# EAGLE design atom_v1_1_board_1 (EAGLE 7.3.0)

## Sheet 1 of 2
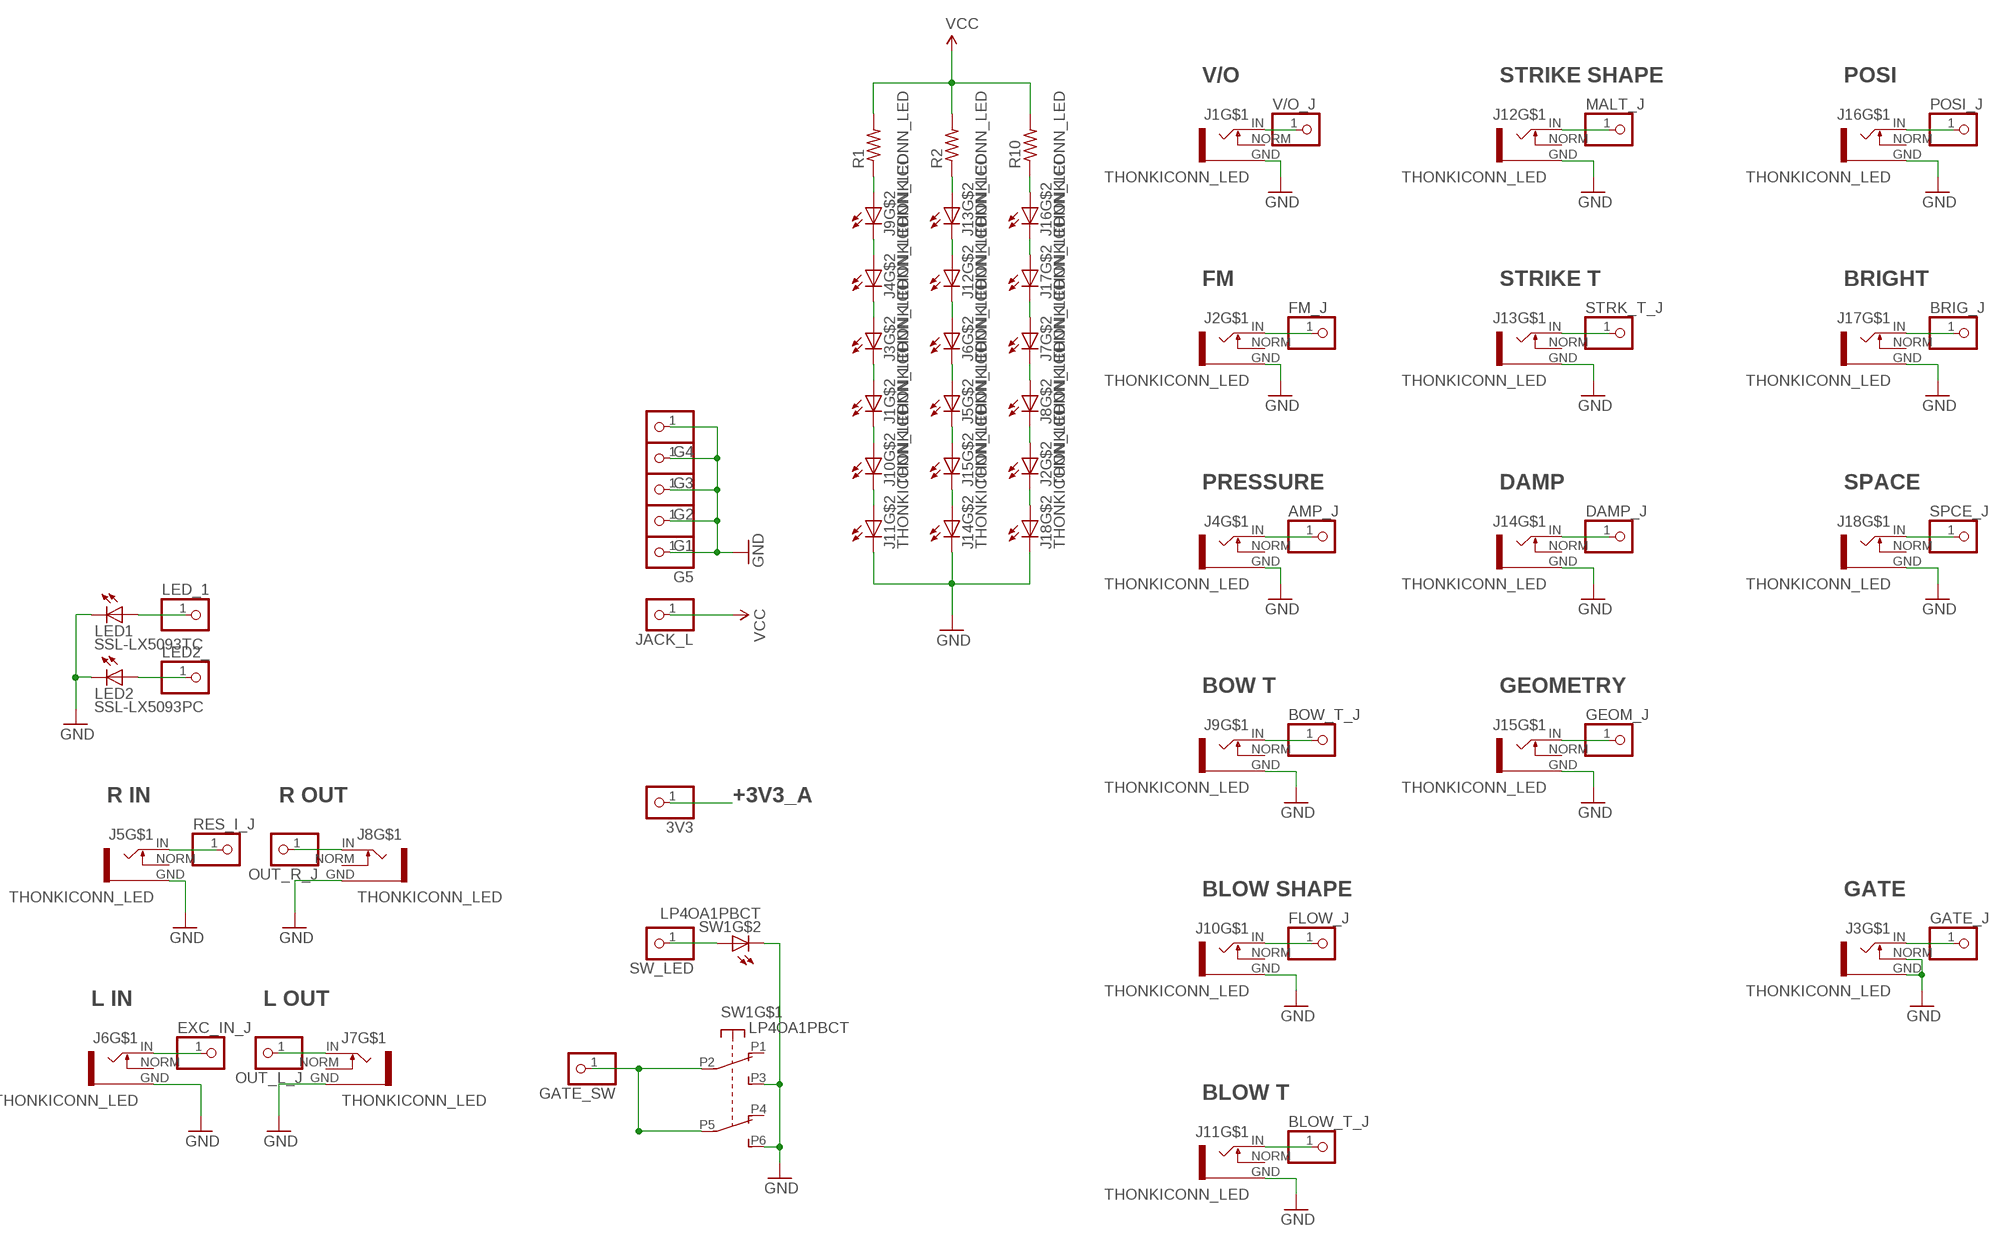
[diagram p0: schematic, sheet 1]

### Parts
3V3  PINHD-1X1  [1X01]
AMP_J  PINHD-1X1  [1X01]
BLOW_T_J  PINHD-1X1  [1X01]
BOW_T_J  PINHD-1X1  [1X01]
BRIG_J  PINHD-1X1  [1X01]
DAMP_J  PINHD-1X1  [1X01]
EXC_IN_J  PINHD-1X1  [1X01]
FLOW_J  PINHD-1X1  [1X01]
FM_J  PINHD-1X1  [1X01]
G1  PINHD-1X1  [1X01]
G2  PINHD-1X1  [1X01]
G3  PINHD-1X1  [1X01]
G4  PINHD-1X1  [1X01]
G5  PINHD-1X1  [1X01]
GATE_J  PINHD-1X1  [1X01]
GATE_SW  PINHD-1X1  [1X01]
GEOM_J  PINHD-1X1  [1X01]
J1  THONKICONN_LED  [LED_JACK]
J2  THONKICONN_LED  [LED_JACK]
J3  THONKICONN_LED  [LED_JACK]
J4  THONKICONN_LED  [LED_JACK]
J5  THONKICONN_LED  [LED_JACK]
J6  THONKICONN_LED  [LED_JACK]
J7  THONKICONN_LED  [LED_JACK]
J8  THONKICONN_LED  [LED_JACK]
J9  THONKICONN_LED  [LED_JACK]
J10  THONKICONN_LED  [LED_JACK]
J11  THONKICONN_LED  [LED_JACK]
J12  THONKICONN_LED  [LED_JACK]
J13  THONKICONN_LED  [LED_JACK]
J14  THONKICONN_LED  [LED_JACK]
J15  THONKICONN_LED  [LED_JACK]
J16  THONKICONN_LED  [LED_JACK]
J17  THONKICONN_LED  [LED_JACK]
J18  THONKICONN_LED  [LED_JACK]
JACK_L  PINHD-1X1  [1X01]
LED1  SSL-LX5093TC  LED5MM  [LED_5MM]
LED2  SSL-LX5093PC  LED5MM  [LED_5MM]
LED2_  PINHD-1X1  [1X01]
LED_1  PINHD-1X1  [1X01]
MALT_J  PINHD-1X1  [1X01]
OUT_L_J  PINHD-1X1  [1X01]
OUT_R_J  PINHD-1X1  [1X01]
POSI_J  PINHD-1X1  [1X01]
R1  RESISTOR  [RESISTOR_0603]
R2  RESISTOR  [RESISTOR_0603]
R10  RESISTOR  [RESISTOR_0603]
RES_I_J  PINHD-1X1  [1X01]
SPCE_J  PINHD-1X1  [1X01]
STRK_T_J  PINHD-1X1  [1X01]
SW1  LP4OA1PBCT  [LP4OA1PBCT]
SW_LED  PINHD-1X1  [1X01]
V/O_J  PINHD-1X1  [1X01]

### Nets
+3V3_A: 3V3.1 ; also sheet 2
GND: G1.1 G2.1 G3.1 G4.1 G5.1 J1.GND J2.GND J3.GND J3.NORM J4.GND J5.GND J6.GND J7.GND J8.GND J9.GND J10.GND J11.C J11.GND J12.GND J13.GND J14.C J14.GND J15.GND J16.GND J17.GND J18.C J18.GND LED1.K(C) LED2.K(C) SW1.L2 SW1.P3(A3) SW1.P6(B3) ; also sheet 2
N$1: J1.IN V/O_J.1
N$3: J12.IN MALT_J.1
N$4 [wide]: J9.A R1.1
N$5 [wide]: J4.A J9.C
N$6: FM_J.1 J2.IN
N$7 [wide]: J3.A J4.C
N$8 [wide]: J1.A J3.C
N$9 [wide]: J1.C J10.A
N$10 [wide]: J10.C J11.A
N$12: J13.IN STRK_T_J.1
N$13 [wide]: J2.C J18.A
N$14 [wide]: J2.A J8.C
N$15 [wide]: J7.C J8.A
N$16: DAMP_J.1 J14.IN
N$17 [wide]: J7.A J17.C
N$18 [wide]: J16.C J17.A
N$19 [wide]: J16.A R10.1
N$20: J5.IN RES_I_J.1
N$21: EXC_IN_J.1 J6.IN
N$22 [wide]: J13.A R2.1
N$23 [wide]: J12.A J13.C
N$24 [wide]: J6.A J12.C
N$25 [wide]: J5.A J6.C
N$26: AMP_J.1 J4.IN
N$27 [wide]: J5.C J15.A
N$28 [wide]: J14.A J15.C
N$29: J16.IN POSI_J.1
N$34: BRIG_J.1 J17.IN
N$36: GEOM_J.1 J15.IN
N$39: J18.IN SPCE_J.1
N$43: GATE_J.1 J3.IN
N$59: LED1.A LED_1.1
N$60: LED2.A LED2_.1
N$83: J8.IN OUT_R_J.1
N$85: J7.IN OUT_L_J.1
N$90: BOW_T_J.1 J9.IN
N$91: FLOW_J.1 J10.IN
N$92: BLOW_T_J.1 J11.IN
N$128: SW1.L1 SW_LED.1
SW_GATE: GATE_SW.1 SW1.P2(A2) SW1.P5(B2)
VCC [wide]: JACK_L.1 R1.2 R2.2 R10.2
Unconnected: J1.NORM J2.NORM J4.NORM J5.NORM J6.NORM J7.NORM J8.NORM J9.NORM J10.NORM J11.NORM J12.NORM J13.NORM J14.NORM J15.NORM J16.NORM J17.NORM J18.NORM SW1.P1(A1) SW1.P4(B1)

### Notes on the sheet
- V/O | STRIKE SHAPE | POSI
- FM | STRIKE T | BRIGHT
- PRESSURE | DAMP | SPACE
- BOW T | GEOMETRY
- R IN | R OUT
- BLOW SHAPE | GATE
- L IN | L OUT
- BLOW T

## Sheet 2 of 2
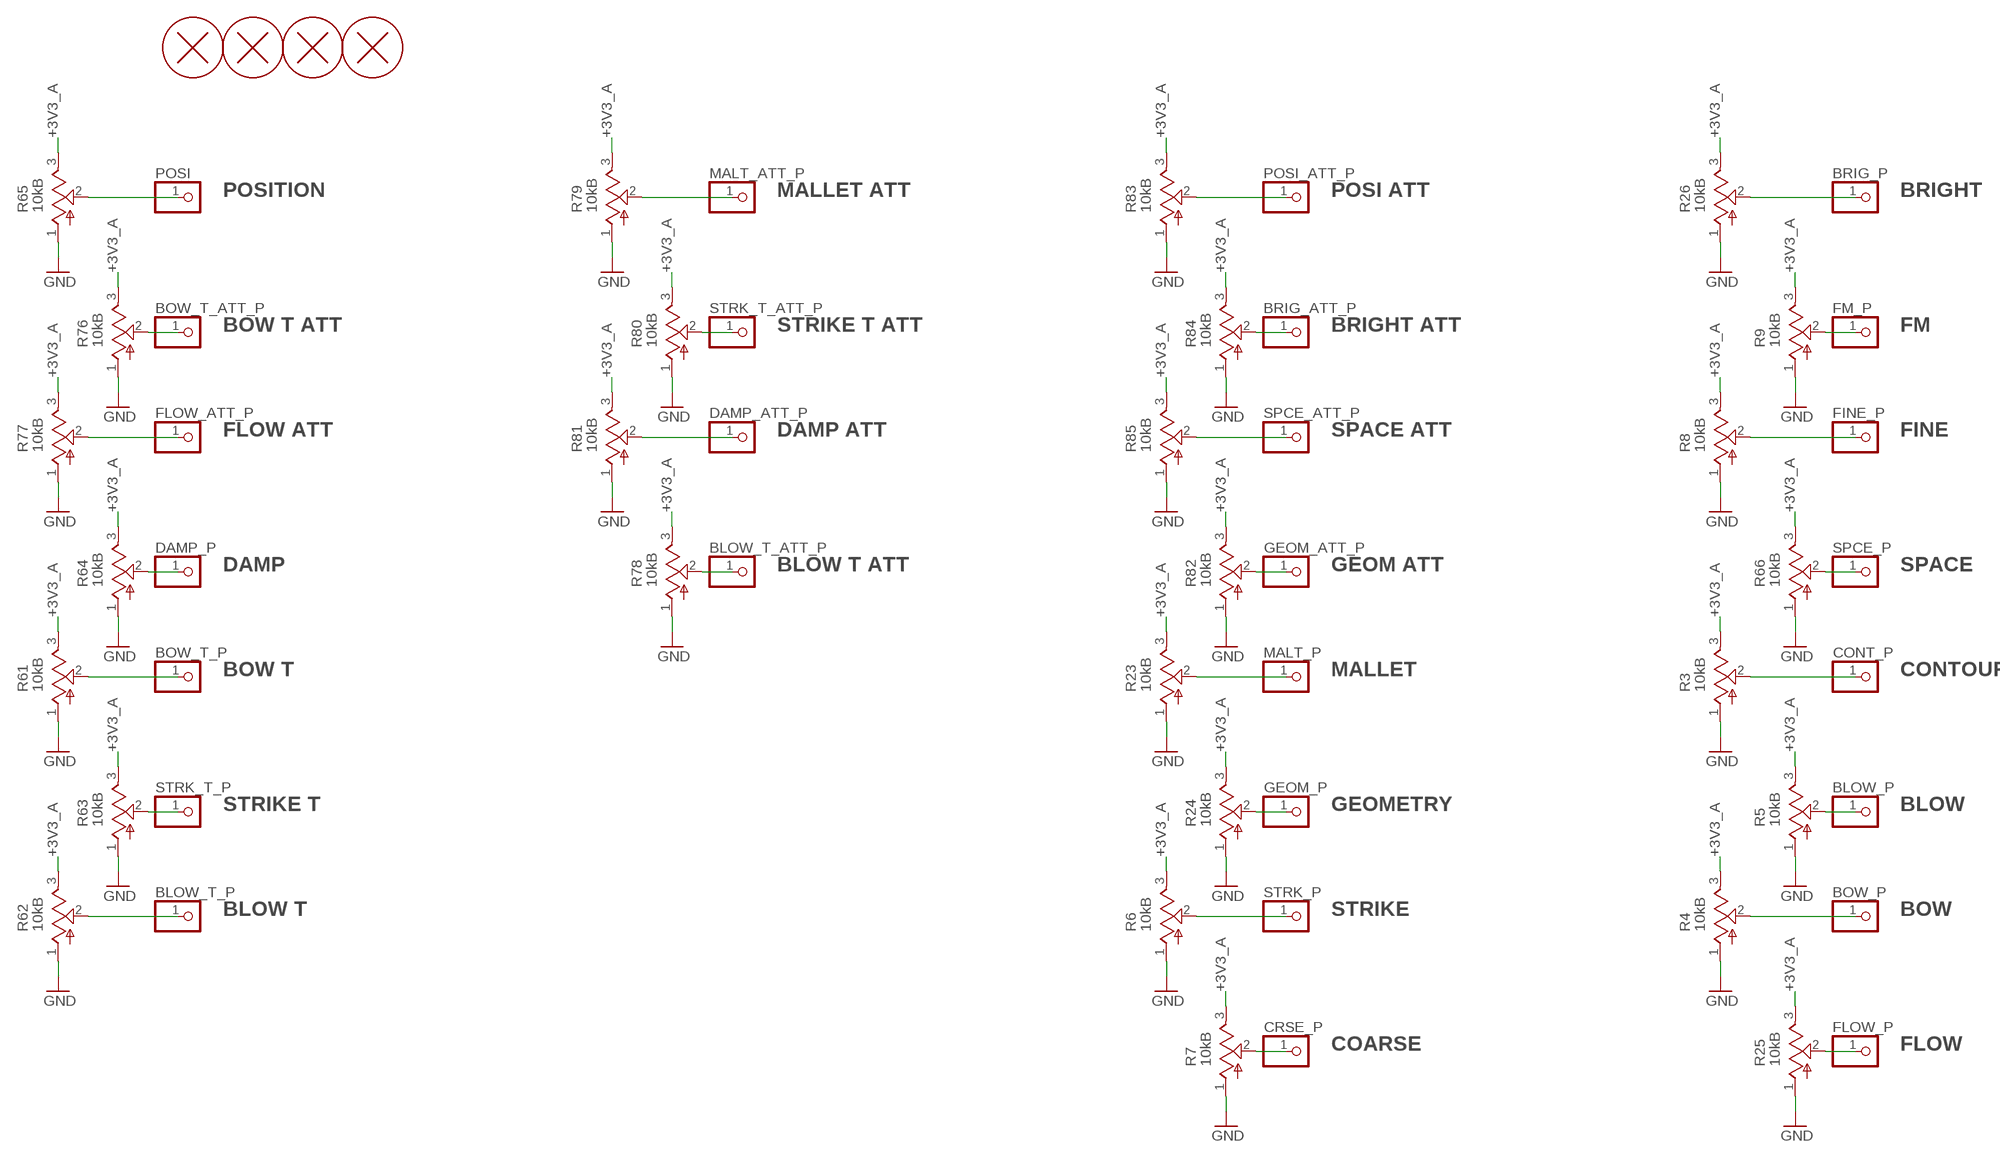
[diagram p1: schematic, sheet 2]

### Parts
BLOW_P  PINHD-1X1  [1X01]
BLOW_T_ATT_P  PINHD-1X1  [1X01]
BLOW_T_P  PINHD-1X1  [1X01]
BOW_P  PINHD-1X1  [1X01]
BOW_T_ATT_P  PINHD-1X1  [1X01]
BOW_T_P  PINHD-1X1  [1X01]
BRIG_ATT_P  PINHD-1X1  [1X01]
BRIG_P  PINHD-1X1  [1X01]
CONT_P  PINHD-1X1  [1X01]
CRSE_P  PINHD-1X1  [1X01]
DAMP_ATT_P  PINHD-1X1  [1X01]
DAMP_P  PINHD-1X1  [1X01]
FINE_P  PINHD-1X1  [1X01]
FLOW_ATT_P  PINHD-1X1  [1X01]
FLOW_P  PINHD-1X1  [1X01]
FM_P  PINHD-1X1  [1X01]
GEOM_ATT_P  PINHD-1X1  [1X01]
GEOM_P  PINHD-1X1  [1X01]
H1  PCB_SCREW  [PCB_SCREW]
H2  PCB_SCREW  [PCB_SCREW]
H3  PCB_SCREW  [PCB_SCREW]
H4  PCB_SCREW  [PCB_SCREW]
MALT_ATT_P  PINHD-1X1  [1X01]
MALT_P  PINHD-1X1  [1X01]
POSI  PINHD-1X1  [1X01]
POSI_ATT_P  PINHD-1X1  [1X01]
R3  10kB  POT_VERTICAL  [ALPS_POT_VERTICAL]
R4  10kB  POT_VERTICAL  [ALPS_POT_VERTICAL]
R5  10kB  POT_VERTICAL  [ALPS_POT_VERTICAL]
R6  10kB  POT_VERTICAL  [ALPS_POT_VERTICAL]
R7  10kB  POT_VERTICAL  [ALPS_POT_VERTICAL]
R8  10kB  POT_VERTICAL  [ALPS_POT_VERTICAL]
R9  10kB  POT_VERTICAL  [ALPS_POT_VERTICAL]
R23  10kB  POT_VERTICAL  [ALPS_POT_VERTICAL]
R24  10kB  POT_VERTICAL  [ALPS_POT_VERTICAL]
R25  10kB  POT_VERTICAL  [ALPS_POT_VERTICAL]
R26  10kB  POT_VERTICAL  [ALPS_POT_VERTICAL]
R61  10kB  POT_VERTICAL  [ALPS_POT_VERTICAL]
R62  10kB  POT_VERTICAL  [ALPS_POT_VERTICAL]
R63  10kB  POT_VERTICAL  [ALPS_POT_VERTICAL]
R64  10kB  POT_VERTICAL  [ALPS_POT_VERTICAL]
R65  10kB  POT_VERTICAL  [ALPS_POT_VERTICAL]
R66  10kB  POT_VERTICAL  [ALPS_POT_VERTICAL]
R76  10kB  POT_VERTICAL  [ALPS_POT_VERTICAL]
R77  10kB  POT_VERTICAL  [ALPS_POT_VERTICAL]
R78  10kB  POT_VERTICAL  [ALPS_POT_VERTICAL]
R79  10kB  POT_VERTICAL  [ALPS_POT_VERTICAL]
R80  10kB  POT_VERTICAL  [ALPS_POT_VERTICAL]
R81  10kB  POT_VERTICAL  [ALPS_POT_VERTICAL]
R82  10kB  POT_VERTICAL  [ALPS_POT_VERTICAL]
R83  10kB  POT_VERTICAL  [ALPS_POT_VERTICAL]
R84  10kB  POT_VERTICAL  [ALPS_POT_VERTICAL]
R85  10kB  POT_VERTICAL  [ALPS_POT_VERTICAL]
SPCE_ATT_P  PINHD-1X1  [1X01]
SPCE_P  PINHD-1X1  [1X01]
STRK_P  PINHD-1X1  [1X01]
STRK_T_ATT_P  PINHD-1X1  [1X01]
STRK_T_P  PINHD-1X1  [1X01]

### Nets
+3V3_A: R3.3(B) R4.3(B) R5.3(B) R6.3(B) R7.3(B) R8.3(B) R9.3(B) R23.3(B) R24.3(B) R25.3(B) R26.3(B) R61.3(B) R62.3(B) R63.3(B) R64.3(B) R65.3(B) R66.3(B) R76.3(B) R77.3(B) R78.3(B) R79.3(B) R80.3(B) R81.3(B) R82.3(B) R83.3(B) R84.3(B) R85.3(B) ; also sheet 1
GND: R3.1(A) R4.1(A) R5.1(A) R6.1(A) R7.1(A) R8.1(A) R9.1(A) R23.1(A) R24.1(A) R25.1(A) R26.1(A) R61.1(A) R62.1(A) R63.1(A) R64.1(A) R65.1(A) R66.1(A) R76.1(A) R77.1(A) R78.1(A) R79.1(A) R80.1(A) R81.1(A) R82.1(A) R83.1(A) R84.1(A) R85.1(A) ; also sheet 1
N$45: BOW_T_ATT_P.1 R76.2(W)
N$46: POSI.1 R65.2(W)
N$47: MALT_ATT_P.1 R79.2(W)
N$48: DAMP_P.1 R64.2(W)
N$49: BOW_T_P.1 R61.2(W)
N$50: R80.2(W) STRK_T_ATT_P.1
N$51: BLOW_T_ATT_P.1 R78.2(W)
N$52: R63.2(W) STRK_T_P.1
N$53: BLOW_T_P.1 R62.2(W)
N$55: FLOW_ATT_P.1 R77.2(W)
N$57: DAMP_ATT_P.1 R81.2(W)
N$58: R85.2(W) SPCE_ATT_P.1
N$62: BRIG_P.1 R26.2(W)
N$63: FINE_P.1 R8.2(W)
N$65: GEOM_ATT_P.1 R82.2(W)
N$67: CRSE_P.1 R7.2(W)
N$68: FM_P.1 R9.2(W)
N$69: R6.2(W) STRK_P.1
N$70: GEOM_P.1 R24.2(W)
N$71: MALT_P.1 R23.2(W)
N$72: FLOW_P.1 R25.2(W)
N$73: BOW_P.1 R4.2(W)
N$74: CONT_P.1 R3.2(W)
N$75: BLOW_P.1 R5.2(W)
N$76: POSI_ATT_P.1 R83.2(W)
N$77: BRIG_ATT_P.1 R84.2(W)
N$78: R66.2(W) SPCE_P.1

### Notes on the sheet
- POSITION | MALLET ATT | POSI ATT | BRIGHT
- BOW T ATT | STRIKE T ATT | BRIGHT ATT | FM
- FLOW ATT | DAMP ATT | SPACE ATT | FINE
- DAMP | BLOW T ATT | GEOM ATT | SPACE
- BOW T | MALLET | CONTOUR
- STRIKE T | GEOMETRY | BLOW
- BLOW T | STRIKE | BOW
- COARSE | FLOW

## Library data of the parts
3V3 AMP_J BLOW_P BLOW_T_ATT_P BLOW_T_J BLOW_T_P BOW_P BOW_T_ATT_P BOW_T_J BOW_T_P BRIG_ATT_P BRIG_J BRIG_P CONT_P CRSE_P DAMP_ATT_P DAMP_J DAMP_P EXC_IN_J FINE_P FLOW_ATT_P FLOW_J FLOW_P FM_J FM_P G1-G5 GATE_J GATE_SW GEOM_ATT_P GEOM_J GEOM_P JACK_L LED2_ LED_1 MALT_ATT_P MALT_J MALT_P OUT_L_J OUT_R_J POSI POSI_ATT_P POSI_J RES_I_J SPCE_ATT_P SPCE_J SPCE_P STRK_P STRK_T_ATT_P STRK_T_J STRK_T_P SW_LED V/O_J = parts_aman:PINHD-1X1: PIN HEADER
H1-H4 = parts_aman:PCB_SCREW
J1-J18 = parts_aman:THONKICONN_LED
LED1 LED2 = parts_aman:LED
R1 R2 R10 = parts_aman:RESISTOR
R3-R9 R23-R26 R61-R66 R76-R85 = parts_aman:POT_VERTICAL
SW1 = og-switch:LP4OA1PBCT

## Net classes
0 default: width 0.152 mm, drill 0.305 mm, clearance 0.152 mm
1 wide: width 0.305 mm, drill 0.305 mm, clearance 0.305 mm

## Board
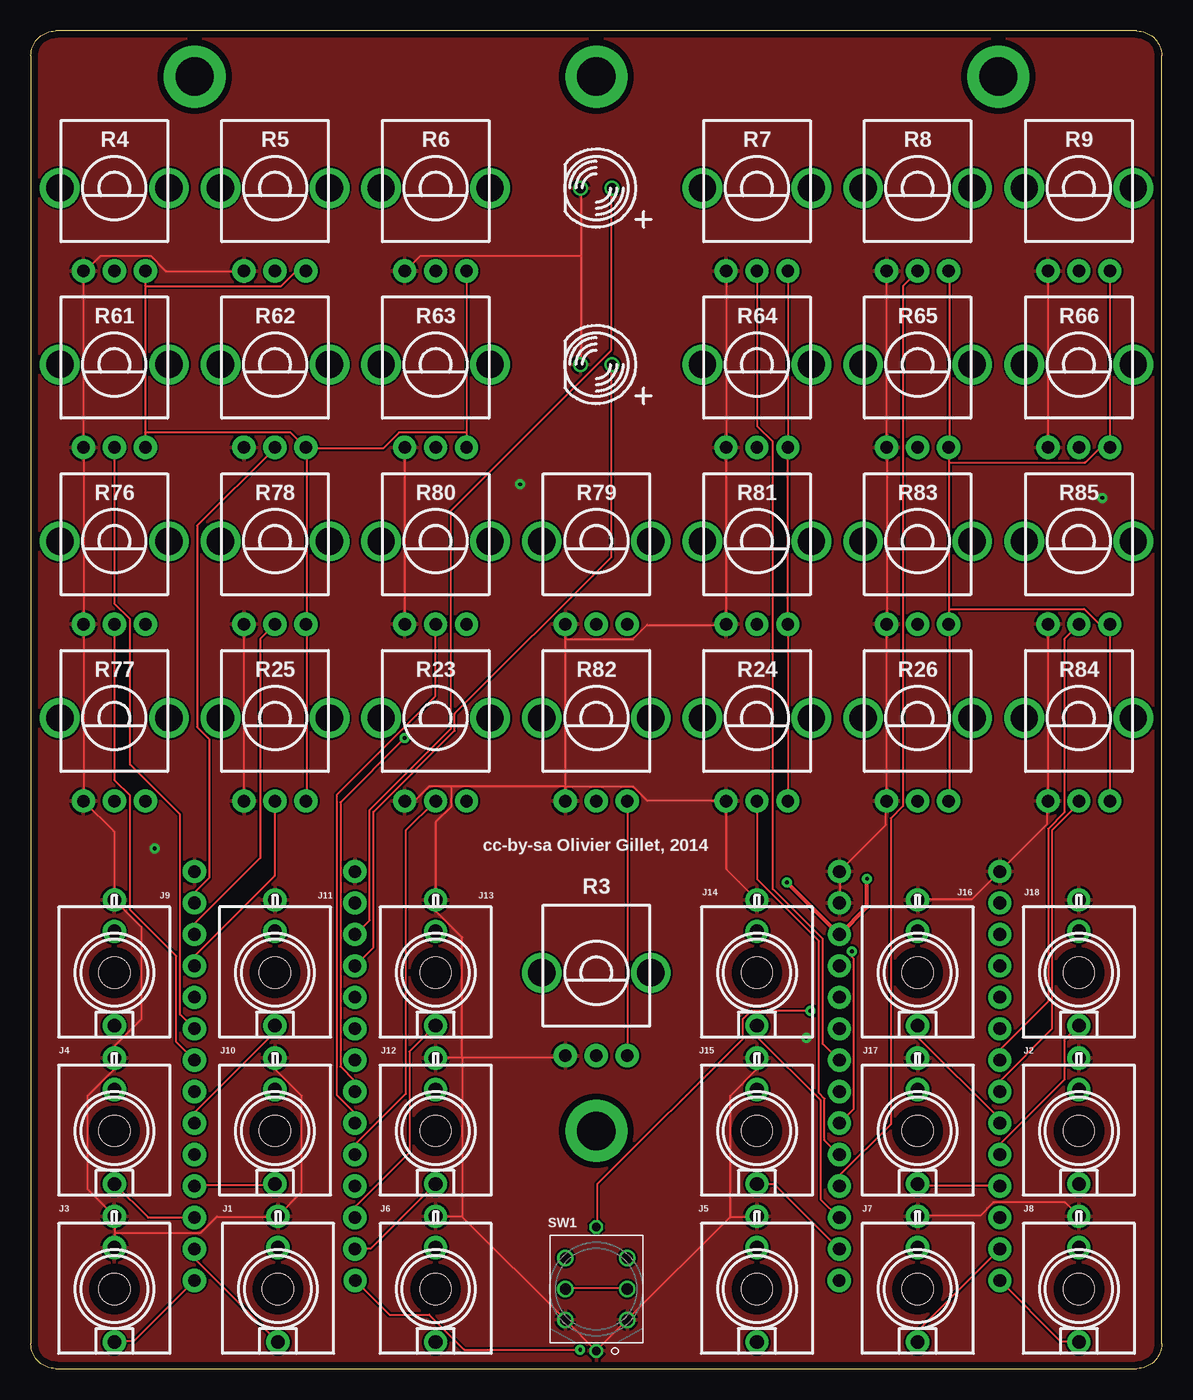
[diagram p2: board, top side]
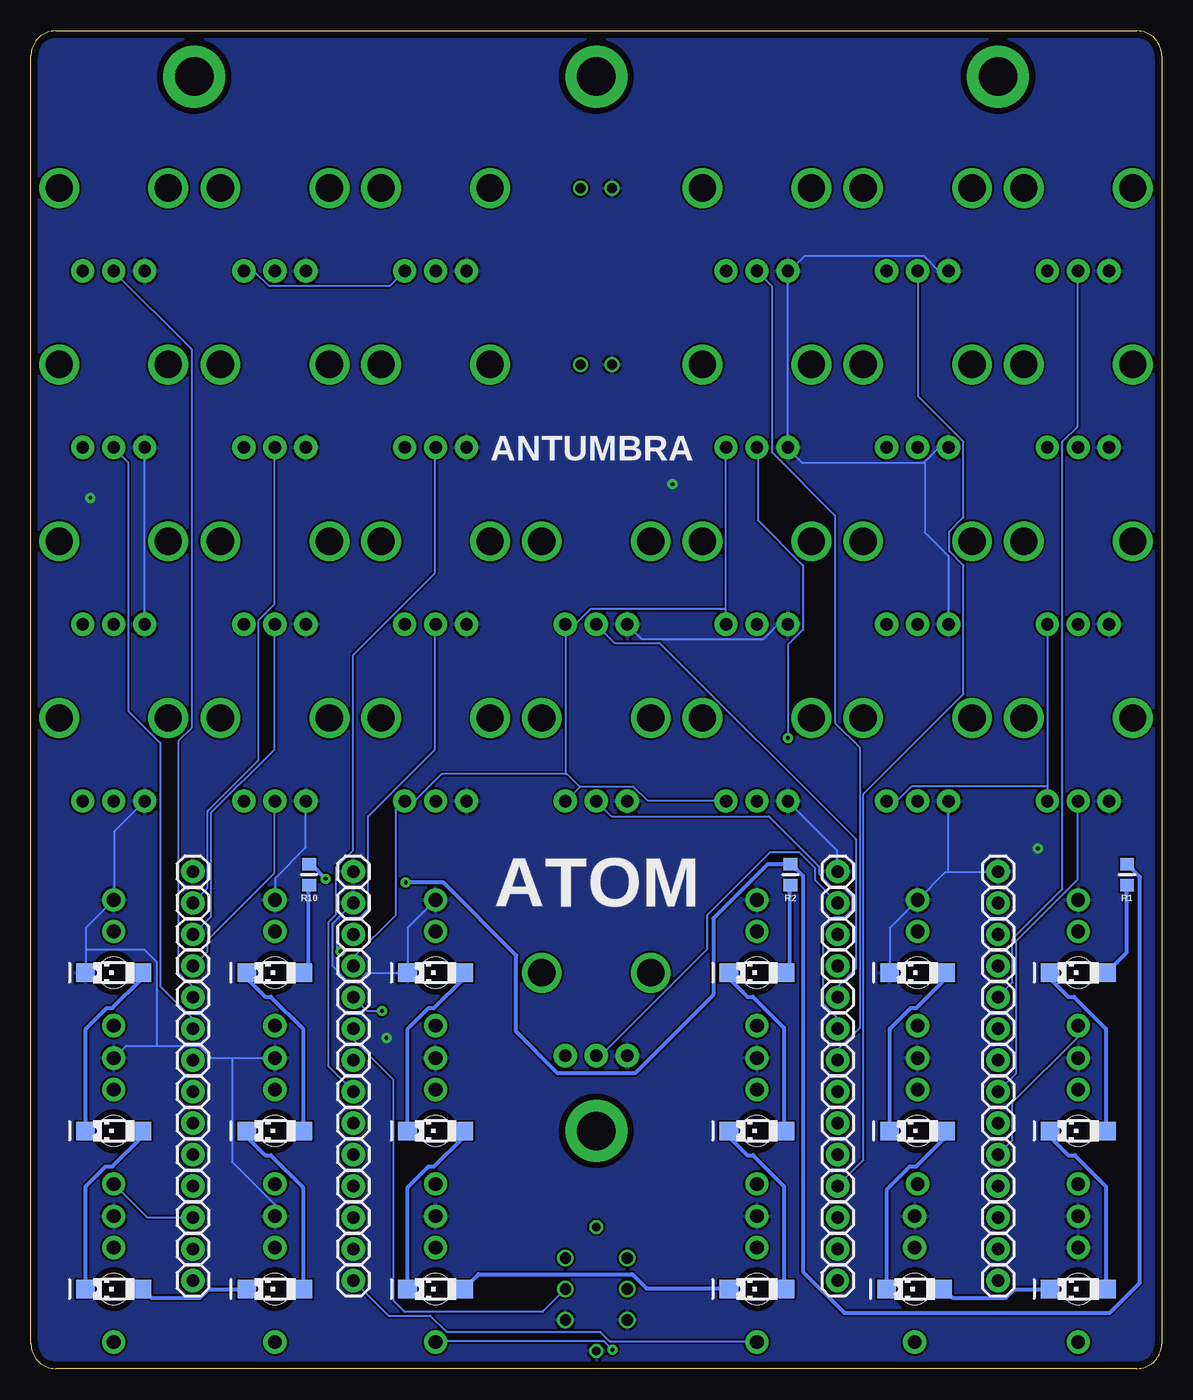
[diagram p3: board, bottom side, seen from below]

Size 91.3 x 108 mm. Coordinates in mm from the lower left corner, seen from the top.
Outline: 2,0 89.3,0 arc90 91.3,2 91.3,106 arc90 89.3,108 2,108 arc90 0,106 0,2 arc90 2,0
Copper layers (1*16): Top 0.035mm / dielectric 1.5mm / Bottom 0.035mm
Design rules "PCBCart-Standard": minimum track width 6mil, minimum drill 12mil, track to track 6mil, track to pad 6mil, pad to pad 6mil, via to via 6mil, smd to smd 6mil, copper to edge 20mil, drill to drill 8mil, minimum pad ring 8mil, minimum via ring 10mil, stop-mask expansion 3mil, vias tented up to drill 25mil, thermal gap 8mil

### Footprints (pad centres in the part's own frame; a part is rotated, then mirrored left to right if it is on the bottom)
1X01 = drill 1.016 pad 1.88: 1 0,0
PCB_SCREW = drill 3.1 pad 5: P$1 0,0
LED_JACK = smd 1.5 x 1.5 bottom: A 2.266,0; C -2.266,0 | drill 1.1 pad 1.88: GND 0,-5.88; IN 0,4.28; NORM 0,-3.34 | hole 2.5: 0,0
LED_5MM = drill 0.813: A -1.27,0; K 1.27,0
RESISTOR_0603 = smd 1 x 1.1: 1 -0.85,0; 2 0.85,0
ALPS_POT_VERTICAL = drill 1 pad 1.88: 1 -2.5,-6.7; 2 0,-6.7; 3 2.5,-6.7 | drill 2.2 pad 3.175: P$4 4.4,0; P$5 -4.4,0
LP4OA1PBCT = drill 0.7 octagon: L1 5,0; L2 -5,0 | drill 0.9: P1 2.5,2.5; P2 0,2.5; P3 -2.5,2.5; P4 2.5,-2.5; P5 0,-2.5; P6 -2.5,-2.5

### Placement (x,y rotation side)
3V3  65.28,32.51 0 bottom
AMP_J  13.21,12.19 0 bottom
BLOW_P  26.16,14.73 0 bottom
BLOW_T_ATT_P  13.21,35.05 0 bottom
BLOW_T_J  13.21,19.81 0 bottom
BLOW_T_P  13.21,37.59 0 bottom
BOW_P  13.21,29.97 0 bottom
BOW_T_ATT_P  13.21,24.89 0 bottom
BOW_T_J  13.21,17.27 0 bottom
BOW_T_P  13.21,27.43 0 bottom
BRIG_ATT_P  78.23,22.35 0 bottom
BRIG_J  78.23,14.73 0 bottom
BRIG_P  78.23,32.51 0 bottom
CONT_P  26.16,37.59 0 bottom
CRSE_P  65.28,24.89 0 bottom
DAMP_ATT_P  65.28,19.81 0 bottom
DAMP_J  65.28,12.19 0 bottom
DAMP_P  65.28,22.35 0 bottom
EXC_IN_J  65.26,7.11 0 bottom
FINE_P  65.28,14.73 0 bottom
FLOW_ATT_P  13.21,22.35 0 bottom
FLOW_J  13.21,14.73 0 bottom
FLOW_P  13.21,32.51 0 bottom
FM_J  78.23,12.19 0 bottom
FM_P  78.23,29.97 0 bottom
G1  13.21,40.13 0 bottom
G2  26.16,40.13 0 bottom
G3  65.28,40.13 0 bottom
G4  78.23,40.13 0 bottom
G5  65.28,37.59 0 bottom
GATE_J  13.21,7.11 0 bottom
GATE_SW  65.28,27.43 0 bottom
GEOM_ATT_P  26.16,27.43 0 bottom
GEOM_J  65.28,9.65 0 bottom
GEOM_P  65.28,17.27 0 bottom
H1  13.22,104.31 0 top
H2  78.12,104.31 0 top
H3  45.65,104.31 0 top
H4  45.65,19.19 0 top
J1  19.94,6.42 180 top
J2  84.62,19.19 180 top
J3  6.74,6.42 180 top
J4  6.74,19.19 180 top
J5  58.62,6.42 180 top
J6  32.68,6.42 180 top
J7  71.6,6.42 180 top
J8  84.62,6.42 180 top
J9  6.74,31.96 180 top
J10  19.7,19.19 180 top
J11  19.7,31.96 180 top
J12  32.68,19.19 180 top
J13  32.68,31.96 180 top
J14  58.62,31.96 180 top
J15  58.62,19.19 180 top
J16  71.6,31.96 180 top
J17  71.6,19.19 180 top
J18  84.62,31.96 180 top
JACK_L  65.28,35.05 0 bottom
LED1  45.65,95.32 180 top
LED2  45.65,81.07 180 top
LED2_  26.16,32.51 0 bottom
LED_1  26.16,35.05 0 bottom
MALT_ATT_P  26.16,29.97 0 bottom
MALT_J  26.16,9.65 0 bottom
MALT_P  26.16,17.27 0 bottom
OUT_L_J  78.23,9.65 0 bottom
OUT_R_J  78.23,7.11 0 bottom
POSI  78.23,37.59 0 bottom
POSI_ATT_P  78.23,35.05 0 bottom
POSI_J  78.23,19.81 0 bottom
R1  2.79,39.88 90 bottom
R2  29.97,39.88 90 bottom
R3  45.65,31.96 0 top
R4  6.74,95.32 0 top
R5  19.7,95.32 0 top
R6  32.68,95.32 0 top
R7  58.62,95.32 0 top
R8  71.6,95.32 0 top
R9  84.62,95.32 0 top
R10  68.83,39.88 90 bottom
R23  32.68,52.52 0 top
R24  58.62,52.52 0 top
R25  19.7,52.52 0 top
R26  71.6,52.52 0 top
R61  6.74,81.07 0 top
R62  19.7,81.07 0 top
R63  32.68,81.07 0 top
R64  58.62,81.07 0 top
R65  71.6,81.07 0 top
R66  84.62,81.07 0 top
R76  6.74,66.8 0 top
R77  6.74,52.52 0 top
R78  19.7,66.8 0 top
R79  45.65,66.8 0 top
R80  32.68,66.8 0 top
R81  58.62,66.8 0 top
R82  45.65,52.52 0 top
R83  71.6,66.8 0 top
R84  84.62,52.52 0 top
R85  84.62,66.8 0 top
RES_I_J  26.18,7.11 0 bottom
SPCE_ATT_P  78.23,24.89 0 bottom
SPCE_J  78.23,17.27 0 bottom
SPCE_P  78.23,27.43 0 bottom
STRK_P  26.16,24.89 0 bottom
STRK_T_ATT_P  26.16,19.81 0 bottom
STRK_T_J  26.16,12.19 0 bottom
STRK_T_P  26.16,22.35 0 bottom
SW1  45.65,6.42 90 top
SW_LED  65.28,29.97 0 bottom
V/O_J  13.21,9.65 0 bottom

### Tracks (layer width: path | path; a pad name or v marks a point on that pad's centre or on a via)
+3V3_A
  Top 0.152: R84.3 87.1,45.87 87.1,60.05 R85.3 87.02,60.05 86.33,60.05 85.04,61.34 74.14,61.34 | R9.3 87.1,88.54 87.1,74.37 R66.3 87.02,74.37 86.33,74.37 85.11,73.15 74.14,73.15 | R8.3 74.14,88.54 74.14,74.37 R65.3 74.14,74.3 74.14,73.15 | R26.3 74.14,45.87 74.14,60.05 R83.3 74.14,60.12 74.14,61.34 | 74.14,61.34 74.14,73.15 | R7.3 61.11,88.54 R64.3 61.11,74.3 61.11,60.12 R81.3 61.11,60.05 61.11,45.87 R24.3 | R3.3 48.16,25.3 48.16,45.8 R82.3 | 9.22,87.4 9.22,88.54 R4.3 | 9.22,87.4 9.22,75.59 | 9.22,75.59 9.22,74.37 R61.3 | 9.22,87.4 20.19,87.4 21.34,88.54 22.17,88.54 R5.3 | R62.3 22.25,74.3 22.25,60.12 R78.3 22.25,60.05 22.25,45.87 R25.3 | 35.2,75.59 35.2,74.37 R63.3 | 35.2,75.59 35.2,88.54 R6.3 | 35.2,75.59 29.72,75.59 28.42,74.3 22.33,74.3 R62.3 | 9.22,75.59 20.95,75.59 22.17,74.37 R62.3
  Bottom 0.152: 3V3.1 65.23,32.54 65.23,33.22 61.87,36.58 61.87,45.11 61.19,45.8 R24.3 61.11,45.87 60.27,45.87 58.14,48.01 48.08,48.01 48.04,48.04 | R8.3 74.07,88.54 73.23,88.54 72.08,87.4 62.33,87.4 61.19,88.54 R7.3 | 46.98,46.98 48.08,45.87 R82.3 | 46.98,46.98 46.94,47.02 42.67,47.02 41.53,45.87 35.2,45.87 R23.3 | 46.98,46.98 48.04,48.04 | 48.04,48.04 48.08,48.08 48.08,60.05 R79.3 48.01,60.05 47.4,60.05 46.1,61.34 35.2,61.34 | 9.22,47.02 9.22,60.05 R76.3 | 9.22,47.02 9.22,45.87 R77.3 | 9.22,47.02 20.19,47.02 21.34,45.87 22.17,45.87 R25.3 | 35.2,61.34 35.2,74.3 R63.3 | 35.2,61.34 35.2,60.12 R80.3
GND  (via drill 0.3)
  Top 0.152: R9.1 82.14,88.54 82.14,74.37 R66.1 | R8.1 69.11,88.54 69.11,74.45 R65.1 69.11,74.3 69.11,60.12 R83.1 69.11,60.05 69.11,45.87 R26.1 69.04,45.8 69.04,43.89 G3.1 65.3,40.08 65.3,37.64 G5.1 | J7.GND 71.63,12.34 76.66,12.34 77.72,13.41 83.52,13.41 84.58,12.34 J8.GND | J14.GND 58.6,37.87 56.16,40.31 56.16,45.8 R24.1 56.08,45.87 49.76,45.87 48.62,47.02 43.13,47.02 | J16.GND 71.63,37.87 75.97,37.87 G4.1 82.07,43.97 82.07,45.8 R84.1 82.14,45.87 82.14,60.05 R85.1 | 6.78,10.97 6.78,12.27 J3.GND 6.71,12.34 4.57,14.48 4.57,22.02 6.71,24.16 6.71,24.99 J4.GND 6.78,25.07 6.78,26.06 8.91,28.19 8.91,35.66 6.78,37.8 J9.GND 6.71,37.87 6.71,43.36 4.27,45.8 R77.1 4.27,45.87 4.27,60.05 R76.1 4.27,60.12 4.27,74.3 R61.1 4.27,74.37 4.27,88.54 R4.1 4.34,88.54 5.64,89.84 9.68,89.84 10.9,88.62 17.14,88.62 R5.1 | 6.78,10.97 6.78,9.83 J3.NORM | 6.78,10.97 13.72,10.97 15.01,12.27 19.89,12.27 J1.GND 19.96,12.34 21.87,14.25 21.87,22.02 19.74,24.16 19.74,24.99 J10.GND | R78.1 17.22,60.05 17.22,45.87 R25.1 | 44.42,89.84 44.42,95.25 LED1.K | 44.42,89.84 44.42,81.08 LED2.K | R80.1 30.18,60.12 30.18,74.3 R63.1 | 44.42,89.84 31.47,89.84 30.25,88.62 R6.1 | 45.64,1.45 43.2,3.89 SW1.P3 43.13,3.96 34.82,12.27 | 45.64,1.45 48.08,3.89 SW1.P6 48.16,3.96 56.46,12.27 | 45.64,1.45 SW1.L2 | 34.82,12.27 32.69,12.27 J6.GND | 56.46,12.27 58.6,12.27 J5.GND | 56.46,12.27 56.46,22.02 58.6,24.16 58.6,24.99 J15.GND | 34.82,25.07 42.98,25.07 43.13,25.22 R3.1 | 34.82,25.07 J12.GND | 34.82,25.07 34.82,34.82 32.69,36.96 32.69,37.8 J13.GND 32.69,37.87 32.69,44.12 33.91,45.34 33.91,47.02 | R7.1 56.16,88.54 56.16,74.37 R64.1 56.16,74.3 56.16,60.12 R81.1 56.08,60.05 49.76,60.05 48.62,58.9 43.13,58.9
  Top 0.152: 43.13,58.9 43.13,60.05 R79.1 | 43.13,58.9 43.13,47.02 | 43.13,47.02 43.13,45.87 R82.1 | 43.13,47.02 33.91,47.02 | 33.91,47.02 32.16,47.02 31.01,45.87 30.25,45.87 R23.1 | 34.82,25.07 34.82,12.27
  Bottom 0.152: R85.1 82.14,60.12 82.14,74.3 R66.1 | 75.06,25.07 76.73,25.07 77.72,26.06 81.15,26.06 | 75.06,25.07 71.63,25.07 J17.GND | 81.15,26.06 83.59,26.06 84.58,25.07 J2.GND | 75.06,25.07 75.06,16.69 71.63,13.26 71.63,12.34 J7.GND | J14.GND 58.67,37.8 60.88,35.59 60.88,32 J14.C 60.96,31.93 64.16,31.93 64.77,31.32 65.76,31.32 66.98,32.54 66.98,35.89 G5.1 | 86.87,33.83 86.87,35.59 84.66,37.8 J18.GND 84.58,37.87 84.58,43.36 82.14,45.8 R84.1 | 86.87,33.83 86.87,32 J18.C | R26.1 69.11,45.8 69.11,42.06 71.55,39.62 71.55,37.87 J16.GND | 81.15,26.06 81.15,32.84 82.14,33.83 86.87,33.83 | J11.C 21.95,32 21.95,35.59 19.74,37.8 J11.GND 19.66,37.87 17.45,40.08 17.22,40.08 | 17.22,40.08 13.26,40.08 G1.1 | 17.22,40.08 17.22,45.8 R25.1 | 19.16,73.19 19.2,73.15 29.03,73.15 30.18,74.3 R63.1 30.18,88.54 R6.1 30.1,88.54 28.8,89.84 19.2,89.84 17.98,88.62 17.22,88.62 R5.1 | 19.16,73.19 18.06,74.3 17.22,74.3 R62.1 | R78.1 17.22,60.12 17.22,65.61 19.13,67.51 19.13,73.15 19.16,73.19 | G2.1 26.21,40.16 26.21,41.83 30.18,45.8 R23.1 | R80.1 30.25,60.05 31.01,60.05 32.16,58.9 41.99,58.9 43.13,60.05 R79.1
  other vias: 39.5,71.4 86.5,70.3 10,42 62.6,26.7
  pour Top: 0,0 91.3,0 91.3,108 0,108
  pour Bottom: 0,0 91.3,0 91.3,108 0,108
N$1
  Top 0.152: V/O_J.1 13.26,9.6 13.26,8.84 19.89,2.21 J1.IN
N$3
  Top 0.152: MALT_J.1 26.21,9.68 27.43,9.68 32.61,14.86 J12.IN
N$4
  Bottom 0.305: R1.1 2.82,39.01 2.82,33.6 4.42,32 J9.A
N$5
  Bottom 0.305: J4.A 4.5,19.2 4.5,27.43 7.09,30.02 7.54,30.02 8.99,31.47 8.99,31.93 J9.C
N$6
  Bottom 0.152: FM_J.1 81.92,12.19 84.58,14.86 J2.IN
N$7
  Bottom 0.305: J3.A 4.5,6.48 4.5,14.71 7.01,17.22 7.54,17.22 8.99,18.67 8.99,19.13 J4.C
N$8
  Bottom 0.305: J3.C 9.07,6.4 11.89,6.4 12.57,5.71 16.92,5.71 17.6,6.4 J1.A
N$9
  Bottom 0.305: J10.A 17.45,19.13 17.45,18.67 19.81,16.31 20.34,16.31 22.17,14.48 22.17,6.48 J1.C
N$10
  Bottom 0.305: J11.A 17.45,31.93 17.45,31.47 19.81,29.11 20.27,29.11 21.95,27.43 21.95,19.2 J10.C
N$12
  Top 0.152: STRK_T_J.1 26.21,12.19 26.21,13.11 30.56,17.45 30.56,25.6 32.61,27.66 J13.IN
N$13
  Bottom 0.305: J18.A 82.37,31.93 82.37,31.47 84.73,29.11 85.19,29.11 86.87,27.43 86.87,19.2 J2.C
N$14
  Bottom 0.305: J2.A 82.37,19.13 82.37,18.67 84.73,16.31 85.27,16.31 86.87,14.71 86.87,6.48 J8.C
N$15
  Bottom 0.305: J7.C 73.91,6.4 76.96,6.4 77.65,5.71 81.61,5.71 82.3,6.4 J8.A
N$16
  Top 0.152: J14.IN 58.67,27.66 58.67,26.75 63.78,21.64 63.78,13.64 65.23,12.19 DAMP_J.1
N$17
  Bottom 0.305: J7.A 69.34,6.48 69.34,14.63 71.93,17.22 72.39,17.22 73.84,18.67 73.84,19.13 J17.C
N$18
  Bottom 0.305: J17.A 69.34,19.2 69.34,27.43 71.93,30.02 72.39,30.02 73.84,31.47 73.84,31.93 J16.C
N$19
  Bottom 0.305: R10.1 68.89,39.01 68.89,32.38 69.27,32 J16.A
N$20  (via drill 0.3)
  Top 0.152: v44.35,1.52 34.98,1.52 32.16,4.34 28.96,4.34 26.21,7.09 RES_I_J.1
  Bottom 0.152: v44.35,1.52 45.03,2.21 58.6,2.21 J5.IN
N$21
  Bottom 0.152: J6.IN 32.69,2.21 44.58,2.21 45.34,2.97 57.76,2.97 59.05,4.27 62.41,4.27 65.23,7.09 EXC_IN_J.1
N$22
  Bottom 0.305: R2.1 30.02,39.01 30.02,32.38 30.4,32 J13.A
N$23
  Bottom 0.305: J12.A 30.48,19.2 30.48,27.51 32.99,30.02 33.45,30.02 34.9,31.47 34.9,31.93 J13.C
N$24
  Bottom 0.305: J6.A 30.48,6.48 30.48,14.71 32.99,17.22 33.45,17.22 34.9,18.67 34.9,19.13 J12.C
N$25
  Bottom 0.305: J6.C 34.98,6.48 41.6,6.48 42.75,7.62 55.17,7.62 56.31,6.48 J5.A
N$26
  Top 0.152: AMP_J.1 9.45,12.19 6.78,14.86 J4.IN
N$27
  Bottom 0.305: J15.A 56.39,19.13 56.39,18.67 58.75,16.31 59.21,16.31 60.88,14.63 60.88,6.48 J5.C
N$28
  Bottom 0.305: J14.A 56.39,31.93 56.39,31.47 58.75,29.11 59.21,29.11 60.88,27.43 60.88,19.2 J15.C
N$29
  Top 0.152: J16.IN 71.63,27.66 71.63,26.75 78.18,20.19 78.18,19.81 POSI_J.1
N$34
  Top 0.152: BRIG_J.1 78.18,14.78 71.7,14.78 71.63,14.86 J17.IN
N$36
  Top 0.152: J15.IN 58.67,14.86 60.05,14.86 65.23,9.68 GEOM_J.1
N$39
  Top 0.152: SPCE_J.1 78.26,17.3 78.26,18.14 83.44,23.32 83.44,26.52 84.58,27.66 J18.IN
N$43
  Top 0.152: GATE_J.1 8.31,2.21 6.78,2.21 J3.IN
N$45
  Top 0.152: BOW_T_ATT_P.1 11.73,26.36 11.73,33.3 8,37.03 8,46.25 6.78,47.47 6.78,60.05 R76.2
N$46
  Bottom 0.152: POSI.1 77.04,38.79 77.04,45.03 72.92,49.15 72.92,60.43 71.63,61.72 71.63,74.3 R65.2
N$47
  Bottom 0.152: MALT_ATT_P.1 26.14,30.02 26.14,30.86 24.69,32.31 24.69,42.75 40.54,58.6 44.2,58.6 45.64,60.05 R79.2
N$48
  Bottom 0.152: R64.2 58.67,74.3 58.67,64.24 65.3,57.61 65.3,41.83 66.67,40.46 66.67,36.65 67.28,36.04 67.28,24.38 65.3,22.4 DAMP_P.1
N$49
  Top 0.152: R61.2 6.78,74.3 6.78,61.72 8,60.5 8,48.77 12.04,44.73 12.04,28.57 13.18,27.43 BOW_T_P.1
N$50
  Top 0.152: STRK_T_ATT_P.1 26.14,19.81 26.14,20.65 24.69,22.1 24.69,46.33 32.61,54.25 32.61,60.05 R80.2
N$51
  Top 0.152: BLOW_T_ATT_P.1 13.26,35.05 13.26,35.97 18.52,41.22 18.52,58.9 19.66,60.05 R78.2
N$52  (via drill 0.3)
  Top 0.152: v30.18,50.9 24.99,45.72 24.99,24.38 26.14,23.24 26.14,22.4 STRK_T_P.1
  Bottom 0.152: v30.18,50.9 30.18,58.45 28.96,59.66 28.96,64.85 32.61,68.5 32.61,74.3 R63.2
N$53
  Top 0.152: BLOW_T_P.1 13.26,37.64 13.26,38.48 14.4,39.62 14.4,50.83 13.41,51.82 13.41,68.05 19.66,74.3 R62.2
N$55
  Bottom 0.152: R77.2 6.78,45.8 6.78,39.47 11.73,34.52 11.73,23.85 13.18,22.4 FLOW_ATT_P.1
N$57  (via drill 0.3)
  Top 0.152: v66.29,33.68 66.29,33.22 66.45,33.07 66.45,20.95 65.3,19.81 DAMP_ATT_P.1
  Bottom 0.152: v66.29,33.68 66.6,33.98 66.6,35.66 65.84,36.42 64.77,36.42 64.08,37.11 64.08,44.58 58.67,49.99 58.67,60.05 R81.2
N$58
  Top 0.152: SPCE_ATT_P.1 78.26,24.92 78.26,25.76 82.14,29.64 82.14,43.59 83.44,44.88 83.44,58.9 84.58,60.05 R85.2
N$59
  Top 0.152: LED1.A 46.86,95.25 46.86,82.22 33.91,69.27 33.91,51.66 27.36,45.11 27.36,36.2 26.21,35.05 LED_1.1
N$60
  Top 0.152: LED2.A 46.86,81 46.86,65.53 34.21,52.88 34.21,51.51 27.66,44.96 27.66,33.98 26.21,32.54 LED2_.1
N$62
  Bottom 0.152: R26.2 71.63,45.8 71.63,40.01 77.04,34.59 77.04,33.68 78.18,32.54 BRIG_P.1
N$63
  Top 0.152: FINE_P.1 65.3,14.78 65.3,15.62 69.42,19.74 69.42,44.42 70.41,45.41 70.41,87.4 71.55,88.54 R8.2
N$65
  Bottom 0.152: GEOM_ATT_P.1 26.21,27.43 26.21,28.35 27.36,29.49 27.36,35.59 26.52,36.42 25.6,36.42 24.99,37.03 24.99,38.1 25.83,38.94 26.67,38.94 27.66,39.93 27.66,40.54 31.7,44.58 44.42,44.58 45.64,45.8 R82.2
N$67
  Top 0.152: R7.2 58.67,88.54 58.67,76.05 59.89,74.83 59.89,38.71 63.93,34.67 63.93,26.21 65.23,24.92 CRSE_P.1
N$68
  Bottom 0.152: FM_P.1 78.26,30.02 78.26,30.86 79.4,32 79.4,50.67 78.33,51.74 78.33,82.3 84.58,88.54 R9.2
N$69
  Bottom 0.152: STRK_P.1 26.14,24.92 26.14,25.76 24.38,27.51 24.38,50.14 26.36,52.12 26.36,68.89 31.47,73.99 31.47,87.4 32.61,88.54 R6.2
N$70
  Top 0.152: R24.2 58.67,45.8 58.67,39.47 63.63,34.52 63.63,22.25 64.08,21.79 64.08,18.44 65.23,17.3 GEOM_P.1
N$71
  Top 0.152: MALT_P.1 26.21,17.3 26.21,18.14 30.25,22.17 30.25,43.43 32.61,45.8 R23.2
N$72
  Top 0.152: FLOW_P.1 13.26,32.54 13.26,33.38 19.66,39.78 19.66,45.8 R25.2
N$73
  Bottom 0.152: R4.2 6.78,88.54 6.78,76.05 8,74.83 8,38.71 12.04,34.67 12.04,31.17 13.18,30.02 BOW_P.1
N$74
  Bottom 0.152: CONT_P.1 27.96,39.4 27.96,40.39 29.26,41.68 31.62,41.68 36.73,36.58 36.73,33.83 45.26,25.3 45.64,25.3 R3.2
N$75
  Bottom 0.152: R5.2 19.66,88.54 19.66,78.49 16,74.83 16,68.73 17.14,67.59 17.14,65.99 16,64.85 16,54.48 24.08,46.41 24.08,16.84 26.14,14.78 BLOW_P.1
N$76
  Bottom 0.152: R83.2 71.63,60.05 71.63,49.99 76.73,44.88 76.73,36.5 78.18,35.05 POSI_ATT_P.1
N$77
  Top 0.152: BRIG_ATT_P.1 78.26,22.4 78.26,23.24 82.45,27.43 82.45,43.43 84.58,45.57 84.58,45.8 R84.2
N$78
  Bottom 0.152: SPCE_P.1 78.26,27.43 78.26,28.27 80.85,30.86 80.85,50.52 83.44,53.11 83.44,73.15 84.58,74.3 R66.2
N$83
  Top 0.152: OUT_R_J.1 83.13,2.21 84.58,2.21 J8.IN
N$85
  Top 0.152: OUT_L_J.1 71.63,3.05 71.63,2.21 J7.IN
N$90
  Bottom 0.152: BOW_T_J.1 12.04,18.44 12.04,21.49 6.78,26.75 6.78,27.66 J9.IN
N$91
  Top 0.152: FLOW_J.1 13.26,14.78 19.58,14.78 19.66,14.86 J10.IN
N$92
  Top 0.152: BLOW_T_J.1 13.26,19.81 13.26,20.73 19.66,27.13 19.66,27.66 J11.IN
N$128  (via drill 0.3)
  Top 0.152: v62.94,28.88 58.14,28.88 57.45,28.19 57.45,26.59 45.72,14.86 45.72,11.43 SW1.L1
  Bottom 0.152: v62.94,28.88 64.16,28.88 65.23,29.95 SW_LED.1
SW_GATE
  Top 0.152: SW1.P2 43.2,6.48 48.08,6.48 SW1.P5
  Bottom 0.152: GATE_SW.1 65.23,27.43 65.23,26.52 62.03,23.32 62.03,5.49 61.11,4.57 49.99,4.57 48.16,6.4 SW1.P5
VCC  (via drill 0.3)
  Top 0.305: v67.51,39.55 67.51,37.26 65.3,35.05 JACK_L.1 65.15,35.13 v61.04,39.24
  Bottom 0.305: v67.51,39.55 68.66,40.69 68.81,40.69 R10.2 | R1.2 2.74,40.69 1.75,39.7 1.75,6.93 4.19,4.5 25.63,4.5 28.96,7.83 28.96,39.78 29.95,40.77 R2.2 30.1,40.69 31.85,40.69 36.2,36.35 36.2,30.18 42.52,23.85 48.77,23.85 52.12,27.2 52.12,33.38 57.99,39.24 v61.04,39.24

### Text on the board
bPlace: ANTUMBRA | ATOM
tNames: cc-by-sa Olivier Gillet, 2014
